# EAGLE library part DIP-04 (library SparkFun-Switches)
4-Position DIP Switch 4-circuit DIP (dual inline package) switch. Commonly used to physcially set a circuit's behavior. SparkFun Products Prototype Part
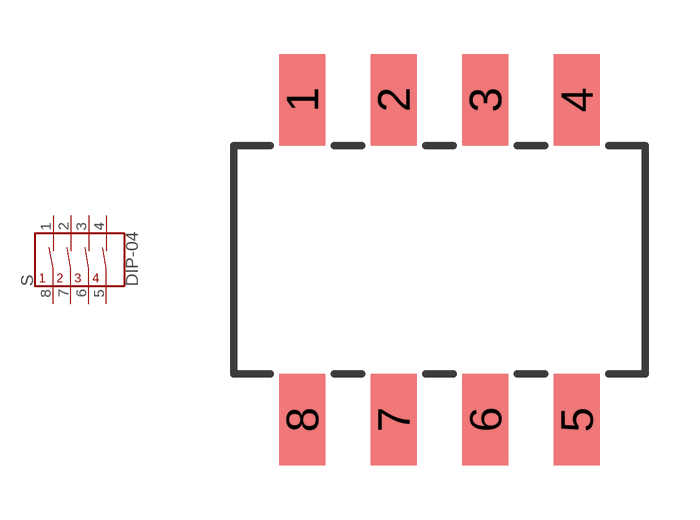
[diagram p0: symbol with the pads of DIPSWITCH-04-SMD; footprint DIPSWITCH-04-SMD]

Designator prefix S

## DIP-04SMD (PROD_ID: SWCH-12418)  [DIPSWITCH-04-SMD]
1  1A
2  2A
3  3A
4  4A
5  4B
6  3B
7  2B
8  1B

## Footprint DIPSWITCH-04-SMD (pad centres in mm)
4-Position DIP Switch - SMD, 0.1"-Pitch Datasheet (219-4MST)
smd 1.27 x 2.54: 1 -3.81,4.445; 2 -1.27,4.445; 3 1.27,4.445; 4 3.81,4.445; 5 3.81,-4.445; 6 1.27,-4.445; 7 -1.27,-4.445; 8 -3.81,-4.445

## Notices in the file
Licensing: Creative Commons ShareAlike 4.0 International - https://creativecommons.org/licenses/by-sa/4.0
